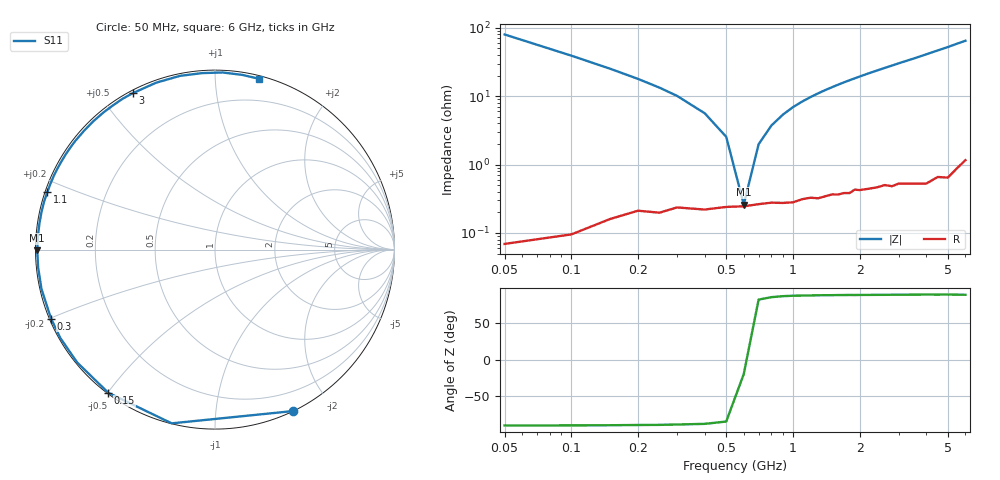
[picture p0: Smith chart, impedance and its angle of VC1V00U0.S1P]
! Infineon Technologies  Discrete & RF Semiconductors
! BBY 56-03
! Si Tuning Diode in SOD323
! VR = 1 V
! S-Parameters:  June  1999
# GHz  S  MA  R  50
!  f  S11
! GHz  MAG  ANG
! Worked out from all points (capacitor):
!   34 points, 50 MHz to 6 GHz, reference 50 ohm
!   read as one part to ground: C = 39.7 pF near 50 MHz
!   lowest |Z| = 260 mohm at 600 MHz (marker M1)
!   series resonance near 604.3 MHz, so ESL is about 1.7 nH
!   S11 on the Smith chart (normalised r, x): 50 MHz: 0.00, -1.59; 150 MHz: 0.00, -0.50; 300 MHz: 0.00, -0.20; 1.1 GHz: 0.01, +0.17; 3 GHz: 0.01, +0.60; 6 GHz: 0.02, +1.29
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0.05  0.9992 -64.2
0.1  0.9976 -104.0
0.15  0.9949 -126.7
0.2  0.9925 -140.7
0.25  0.9926 -150.2
0.3  0.991 -157.2
0.4  0.9914 -167.2
0.5  0.9905 -174.2
0.6  0.9902 -179.8
0.7  0.9895 175.5
0.8  0.989 171.5
1  0.9891 164.3
1.1  0.988 161.1
1.3  0.9878 155.2
1.4  0.9871 152.4
1.6  0.9867 147.2
1.8  0.9864 142.3
2  0.9854 137.7
2.2  0.9852 133.3
2.4  0.9849 129.2
2.6  0.9843 125.2
3  0.9847 117.8
3.5  0.9861 109.4
4  0.9875 101.4
4.5  0.986 94.1
5  0.9878 87.5
5.5  0.9852 81.1
6  0.9828 75.6
